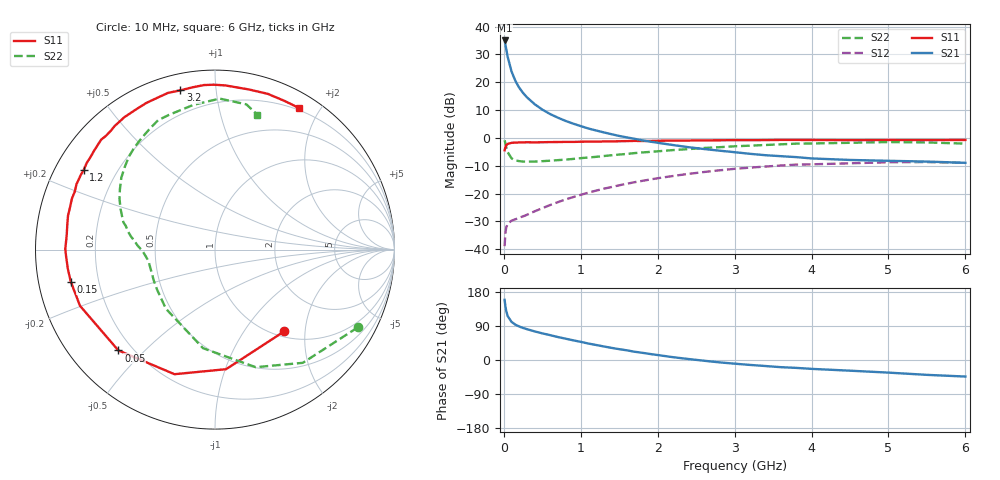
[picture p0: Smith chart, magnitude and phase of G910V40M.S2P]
! SIEMENS Small Signal Semiconductors
! BFG235
! Si NPN RF Bipolar Junction Transistor in SOT223
! VCE = 10 V  IC = 40 mA
! Common Emitter S-Parameters:  July  1994
# GHz  S  MA  R  50
!  f  S11  S21  S12  S22
! GHz  MAG  ANG  MAG  ANG  MAG  ANG  MAG  ANG
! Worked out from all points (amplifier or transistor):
!   40 points, 10 MHz to 6 GHz, reference 50 ohm
!   highest |S21| = 35.0 dB at 10 MHz (marker M1)
!   |S21| within 3 dB of that: start of sweep to 30.49 MHz
!   unconditionally stable (mu >= 1): 540.2 MHz to 1.292 GHz
!   at 200 MHz: K = 0.60, MSG = 23.4 dB, |S12| = -28.7 dB
!   at 1.5 GHz: K = 0.97, MSG = 8.9 dB, |S12| = -17.1 dB
!   at 6 GHz: K = 0.94, MSG = 0.0 dB, |S12| = -9.0 dB
!   S11 on the Smith chart (normalised r, x): 10 MHz: 1.10, -1.56; 50 MHz: 0.15, -0.42; 150 MHz: 0.10, -0.11; 1.2 GHz: 0.08, +0.28; 3.2 GHz: 0.08, +0.80; 6 GHz: 0.18, +1.75
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0.01  0.5971 -49.6  56.42 158.9  0.0113 71.3  0.9057 -28.6
0.02  0.6691 -84.7  47.88 142.3  0.0191 55.2  0.7984 -52.2
0.03  0.73 -108.0  40.28 130.3  0.0242 45.3  0.6933 -70.9
0.05  0.7781 -133.8  28.49 115.8  0.0287 34.8  0.5534 -96.9
0.1  0.8148 -157.4  15.64 100.6  0.0325 28.5  0.4282 -129.7
0.15  0.8232 -167.5  10.6 93.2  0.0344 30.4  0.3925 -145.2
0.2  0.827 -172.7  7.968 88.4  0.0368 33.1  0.3817 -153.8
0.25  0.8298 -176.9  6.418 84.5  0.0388 36.3  0.3754 -159.2
0.3  0.8343 179.8  5.37 81.4  0.0414 39.3  0.3747 -163.5
0.4  0.83 174.8  4.036 75.5  0.0478 44.3  0.3751 -168.5
0.5  0.8344 170.5  3.225 70.3  0.0544 48.4  0.381 -172.1
0.6  0.8405 167.0  2.687 65.7  0.0619 50.9  0.3886 -174.8
0.7  0.8417 163.3  2.315 60.7  0.0697 52.8  0.3976 -177.3
0.9  0.8454 157.6  1.805 52.0  0.0861 54.3  0.4183 178.9
1.1  0.8554 151.0  1.473 43.4  0.1036 54.4  0.444 175.0
1.2  0.8557 148.7  1.357 39.6  0.1127 54.0  0.4564 173.2
1.7  0.8818 136.0  0.962 21.8  0.1597 48.7  0.5326 163.4
2.2  0.894 124.4  0.743 7.4  0.2065 40.5  0.6032 151.9
3.2  0.9079 102.3  0.517 -13.0  0.2918 20.3  0.7245 128.4
4.5  0.9119 78.1  0.401 -28.2  0.349 -6.8  0.8155 98.4
5.5  0.9145 64.9  0.375 -39.2  0.367 -25.9  0.8278 77.8
6  0.9172 59.2  0.356 -43.7  0.3548 -32.8  0.7883 72.7
